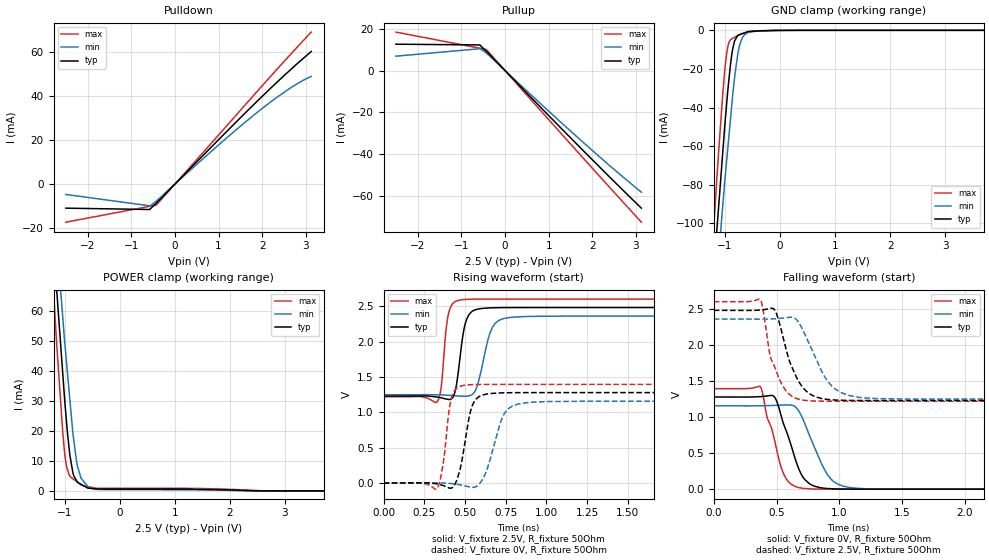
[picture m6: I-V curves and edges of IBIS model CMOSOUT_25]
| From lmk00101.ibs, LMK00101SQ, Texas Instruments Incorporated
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|   Model CMOSOUT_25
[Model]   CMOSOUT_25
Model_type   3-state
Polarity   Non-Inverting
Vmeas = 1.25
Vref = 1.25
Cref = 15pF
Rref = 50
|   typ   min   max
|   Nom   Strong   Weak
C_comp   0.4977p   0.4681p   0.5375p
|Output in High
|C_Comp high   0.4977p   0.4681p   0.5375p
|Output in low
|C_Comp low   0.9197p   0.9197p   0.9197p
|Output disabled
|C_Comp disabled   0.8920p   0.8648p   0.9197p
[Voltage Range]   2.5   2.375   2.625
[Temperature Range]   45   125   -40
[Pullup Reference]   2.5   2.375   2.625
[Pulldown Reference]   0   0   0
[Power Clamp Reference]   2.5   2.375   2.625
[GND Clamp Reference]   0   0   0
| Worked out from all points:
|   slope of the pulldown table from 0 to 0.375 V, typ, clamps not added: 49.4 ohm
|   slope of the pullup table from 0 to 0.375 V, typ, clamps not added: 46.2 ohm
|   GND clamp passes 1 mA (typ) near -0.61 V on its own axis
|   POWER clamp passes 1 mA (typ) near -0.59 V on its own axis
|   falling waveform, V_fixture 0V, R_fixture 50Ohm: 20-80 % time 148ps typ, 175ps min, 130ps max; typ from 1.28 V to 0 V
|   rising waveform, V_fixture 2.5V, R_fixture 50Ohm: 20-80 % time 45.8ps typ, 69.9ps min, 33ps max; typ from 1.23 V to 2.48 V
|   rising waveform, V_fixture 0V, R_fixture 50Ohm: 20-80 % time 59.1ps typ, 88.5ps min, 42.4ps max; typ from 0 V to 1.28 V
|   falling waveform, V_fixture 2.5V, R_fixture 50Ohm: 20-80 % time 148ps typ, 191ps min, 123ps max; typ from 2.48 V to 1.23 V
[Pulldown]
|   Voltage   I(typ)   I(min)   I(max)
-2.5V     -10.91mA   -4.684mA   -17.29mA
-578mV    -11.53mA   -9.847mA   -10.09mA
-428.6mV  -8.635mA   -7.742mA   -9.527mA
980.8mV   19.79mA    17.44mA    21.86mA
1.881V    37.59mA    32.5mA     42.03mA
2.331V    46.13mA    39.34mA    51.97mA
2.631V    51.63mA    43.46mA    58.5mA
3.124V    60.24mA    48.93mA    69.06mA
[GND Clamp]
|   Voltage   I(typ)   I(min)   I(max)
-2.5V     -678.4mA   -642.6mA   -732.3mA
-1.294V   -164mA     -182.8mA   -144.6mA
-1.144V   -103.6mA   -128.3mA   -76.8mA
-1.107V   -89.5mA    -115.2mA   -60.76mA
-1.032V   -61.34mA   -89.07mA   -31.21mA
-955.1mV  -34.32mA   -64.07mA   -9.897mA
-903.7mV  -19.47mA   -48.15mA   -5.202mA
-856.8mV  -9.713mA   -33.64mA   -4.135mA
-763.1mV  -2.595mA   -12.22mA   -2.735mA
-644.3mV  -1.324mA   -2.314mA   -1.452mA
-448.3mV  -404.5uA   -280.1uA   -514.5uA
4.992V    0A         0A         0A
[Pullup]
|   Voltage   I(typ)   I(min)   I(max)
-2.5V     12.61mA    6.884mA    18.41mA
-578mV    12.26mA    10.45mA    10.69mA
-428.6mV  9.218mA    8.382mA    10.09mA
1.581V    -33.88mA   -30.45mA   -37.01mA
2.331V    -49.59mA   -44.29mA   -54.38mA
3.124V    -65.86mA   -58.23mA   -72.59mA
[POWER Clamp]
|   Voltage   I(typ)   I(min)   I(max)
-2.5V     462.1mA    438.3mA    498.2mA
-1.294V   108.8mA    121.8mA    95.52mA
-1.151V   69.13mA    85.95mA    51.4mA
-1.144V   67.51mA    84.5mA     49.52mA
-1.032V   39.01mA    57.79mA    19.39mA
-967.9mV  23.81mA    43.66mA    8.455mA
-903.7mV  11.95mA    30.49mA    5.004mA
-847.4mV  5.957mA    19.15mA    4.055mA
-766.2mV  2.958mA    8.319mA    2.916mA
-692.6mV  2.124mA    4.056mA    1.886mA
-448.3mV  745uA      521.9uA    963.4uA
4.992V    0A         0A         0A
[Ramp]
R_load = 50
|   typ   min   max
dV/dt_r   0.752285/4.55517e-11   0.668144/6.88274e-11   0.83006/3.29105e-11
dV/dt_f   0.768538/1.47551e-10   0.695044/1.73531e-10   0.838167/1.30019e-10
[Falling Waveform]
V_fixture = 0V
V_fixture_min = 0V
V_fixture_max = 0V
R_fixture = 50Ohm
C_fixture = 0F
|   Time   V(typ)   V(min)   V(max)
0s        1.281V     1.158V     1.397V
371ps     1.286V     1.159V     1.424V
424ps     1.296V     1.161V     1.006V
480ps     1.289V     1.164V     715.5mV
551ps     932.9mV    1.169V     235.8mV
642ps     462.4mV    1.155V     43.21mV
699ps     202.4mV    1.018V     14.66mV
910ps     8.486mV    192mV      281.5uV
1.092ns   639.1uV    20.89mV    11.59uV
4.999ns   8.709nV    35.41nV    8.985nV
[Rising Waveform]
V_fixture = 2.5V
V_fixture_min = 2.375V
V_fixture_max = 2.625V
R_fixture = 50Ohm
C_fixture = 0F
|   Time   V(typ)   V(min)   V(max)
0s        1.231V     1.25V      1.221V
330ps     1.217V     1.25V      1.154V
353ps     1.207V     1.248V     1.352V
399ps     1.183V     1.242V     2.403V
437ps     1.281V     1.236V     2.566V
480ps     1.983V     1.23V      2.595V
542ps     2.429V     1.25V      2.603V
666ps     2.481V     2.195V     2.605V
784ps     2.484V     2.347V     2.605V
4.999ns   2.485V     2.364V     2.605V
[Rising Waveform]
V_fixture = 0V
V_fixture_min = 0V
V_fixture_max = 0V
R_fixture = 50Ohm
C_fixture = 0F
|   Time   V(typ)   V(min)   V(max)
0s        8.709nV    35.41nV    8.985nV
328ps     -11.61mV   2.93mV     -77.06mV
363ps     -32.69mV   1.628mV    241.9mV
416ps     -71.23mV   -7.19mV    1.201V
468ps     183.3mV    -23.63mV   1.369V
504ps     642mV      -41.35mV   1.387V
583ps     1.219V     -23.36mV   1.396V
742ps     1.278V     987.2mV    1.397V
882ps     1.281V     1.139V     1.397V
4.999ns   1.281V     1.158V     1.397V
[Falling Waveform]
|Gnd
V_fixture = 2.5V
V_fixture_min = 2.375V
V_fixture_max = 2.625V
R_fixture = 50Ohm
C_fixture = 0F
|   Time   V(typ)   V(min)   V(max)
0s        2.485V     2.364V     2.605V
370ps     2.489V     2.363V     2.635V
394ps     2.493V     2.363V     2.483V
450ps     2.512V     2.365V     1.847V
478ps     2.506V     2.367V     1.728V
578ps     1.935V     2.383V     1.363V
711ps     1.411V     2.209V     1.238V
919ps     1.245V     1.475V     1.222V
1.156ns   1.232V     1.276V     1.221V
4.999ns   1.231V     1.25V      1.221V
